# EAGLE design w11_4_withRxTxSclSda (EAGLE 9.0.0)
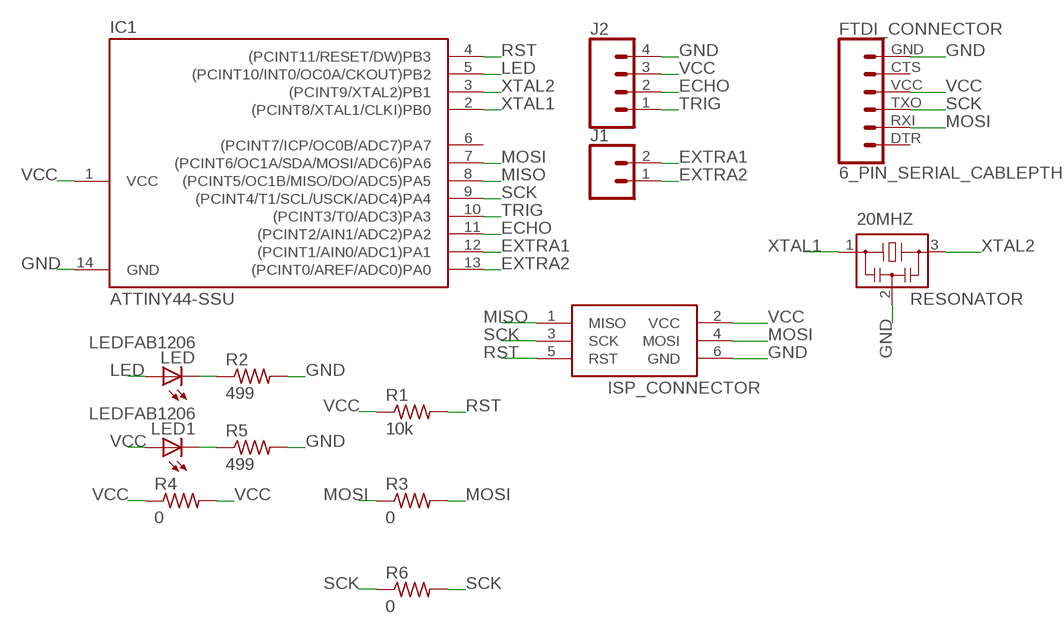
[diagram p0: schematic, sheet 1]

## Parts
20MHZ  RESONATOR  [EFOBM]
FTDI_CONNECTOR  6_PIN_SERIAL_CABLEPTH  [FTDI_BASIC]
IC1  ATTINY44-SSU  [SOIC14]
ISP_CONNECTOR  AVRISP-6  [AVRISP]
J1  CONN_02  [1X02]
J2  CONN_04  [1X04]
LED  LEDFAB1206  [LED1206FAB]
LED1  LEDFAB1206  [LED1206FAB]
R1  10k  RES-US1206FAB  [R1206FAB]
R2  499  RES-US1206FAB  [R1206FAB]
R3  0  RES-US1206FAB  [R1206FAB]
R4  0  RES-US1206FAB  [R1206FAB]
R5  499  RES-US1206FAB  [R1206FAB]
R6  0  RES-US1206FAB  [R1206FAB]

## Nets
ECHO: IC1.11((PCINT2/AIN1/ADC2)PA2) J2.2
EXTRA1: IC1.12((PCINT1/AIN0/ADC1)PA1) J1.2
EXTRA2: IC1.13((PCINT0/AREF/ADC0)PA0) J1.1
GND: 20MHZ.2 FTDI_CONNECTOR.GND IC1.14(GND) ISP_CONNECTOR.6(GND) J2.4 R2.2 R5.2
LED: IC1.5((PCINT10/INT0/OC0A/CKOUT)PB2) LED.1(A)
MISO: IC1.8((PCINT5/OC1B/MISO/DO/ADC5)PA5) ISP_CONNECTOR.1(MISO)
MOSI: FTDI_CONNECTOR.RXI IC1.7((PCINT6/OC1A/SDA/MOSI/ADC6)PA6) ISP_CONNECTOR.4(MOSI) R3.1 R3.2
N$1: LED1.2(C) R5.1
N$5: LED.2(C) R2.1
RST: IC1.4((PCINT11/RESET/DW)PB3) ISP_CONNECTOR.5(RST) R1.2
SCK: FTDI_CONNECTOR.TXO IC1.9((PCINT4/T1/SCL/USCK/ADC4)PA4) ISP_CONNECTOR.3(SCK) R6.1 R6.2
TRIG: IC1.10((PCINT3/T0/ADC3)PA3) J2.1
VCC: FTDI_CONNECTOR.VCC IC1.1(VCC) ISP_CONNECTOR.2(VCC) J2.3 LED1.1(A) R1.1 R4.1 R4.2
XTAL1: 20MHZ.1 IC1.2((PCINT8/XTAL1/CLKI)PB0)
XTAL2: 20MHZ.3 IC1.3((PCINT9/XTAL2)PB1)
Unconnected: FTDI_CONNECTOR.CTS FTDI_CONNECTOR.DTR IC1.6((PCINT7/ICP/OC0B/ADC7)PA7)

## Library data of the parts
20MHZ = fab:RESONATOR
FTDI_CONNECTOR = SparkFun-Connectors:6_PIN_SERIAL_CABLE: 6-pin header connection for use with the "FTDI BASIC" pinout - CABLE SIDE. Also known as "Arduino Serial Program Header". This is used on a design to provide a 6-pin connection point for serial communication usually from a USB cable (D+/D-) to these headers (RX/TX). It also has the remaining pins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
IC1 = fab:ATTINY44
ISP_CONNECTOR = adafruit:AVRISP: AVR ISP HEADER Standard 6 pin header for AVR programming
J1 = SparkFun-Connectors:CONN_02: Multi connection point. Often used as Generic Header-pin footprint for 0.1 inch spaced/style header connections
J2 = SparkFun-Connectors:CONN_04: Multi connection point. Often used as Generic Header-pin footprint for 0.1 inch spaced/style header connections On any of the 0.1 inch spaced packages, you can populate with these: Break Away Headers - Straight (PRT-00116) Break Away Male Headers - Right Angle (PRT-00553) Female Headers (PRT-00115)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; PROD_ID: CONN-09696
LED LED1 = fab:LED: LED
R1-R6 = fab:RES-US: Resistor (US Symbol)

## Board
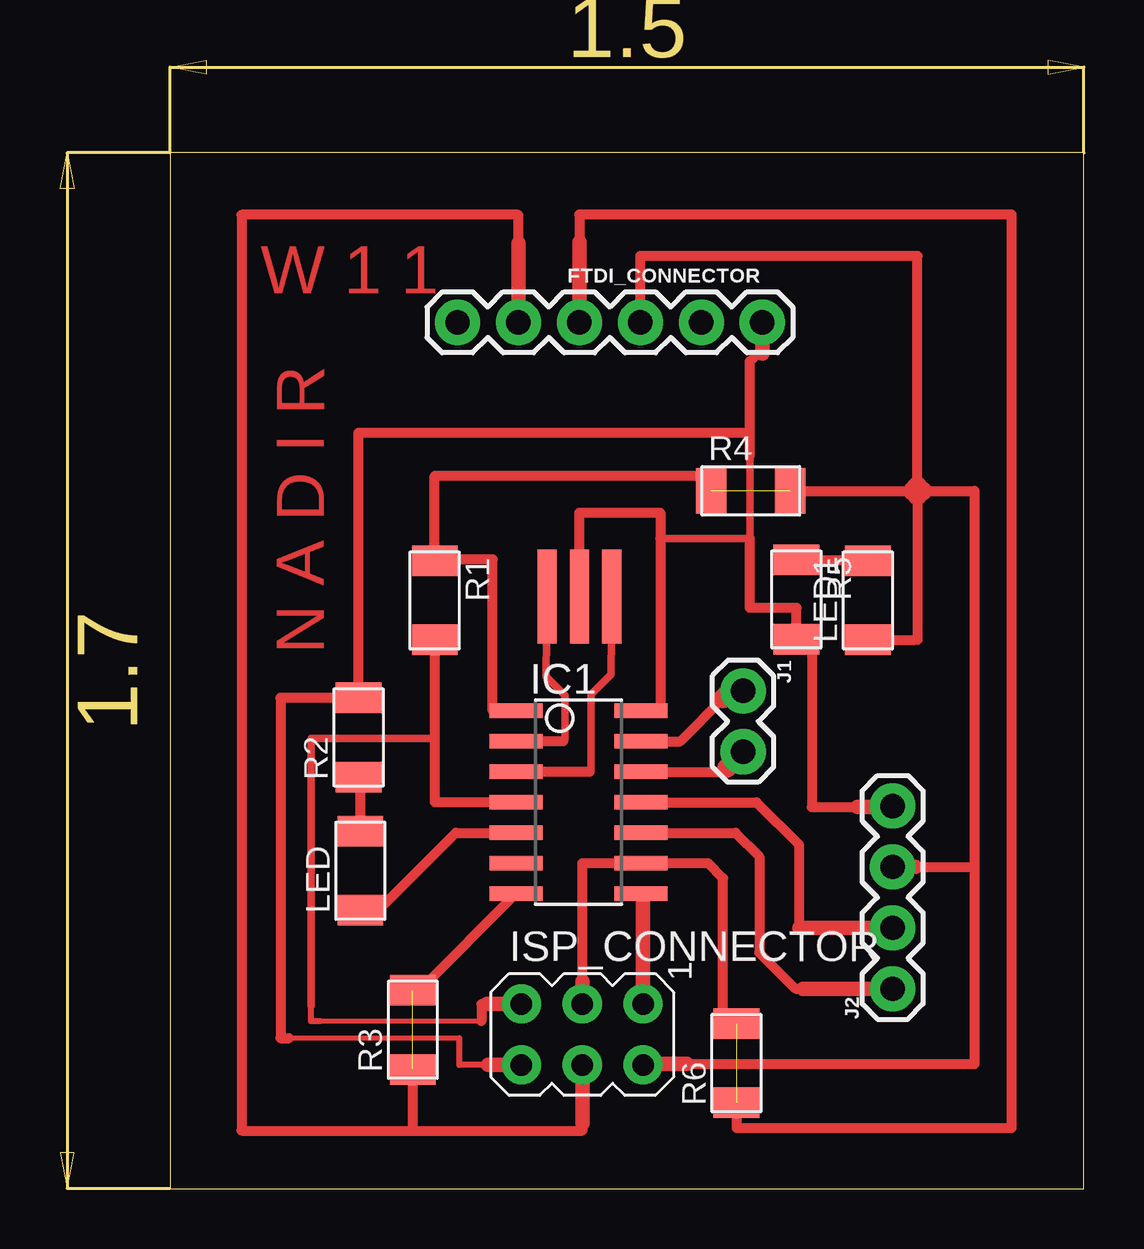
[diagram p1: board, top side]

Size 42.69 x 47.05 mm. Coordinates in mm from the lower left corner, seen from the top.
Outline: 4.59,0 42.69,0 42.69,43.18 4.59,43.18 4.59,0
Copper layers (1*16): Top 0.035mm / dielectric 1.5mm / Bottom 0.035mm
Design rules "default": minimum track width 6mil, minimum drill 0.35mm, track to track 6mil, track to pad 6mil, pad to pad 6mil, via to via 6mil, smd to smd 6mil, copper to edge 40mil, drill to drill 6mil, minimum pad ring 10mil, minimum via ring 8mil, stop-mask expansion 4mil, vias tented up to drill 0mil, thermal gap 10mil

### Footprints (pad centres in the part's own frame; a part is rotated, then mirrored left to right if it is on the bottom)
EFOBM = smd 0.8 x 3.9: 1 -1.35,0; 2 0,0; 3 1.35,0
FTDI_BASIC = drill 1.016 pad 1.88: CTS 10.16,0; DTR 0,0; GND 12.7,0; RXI 2.54,0; TXO 5.08,0; VCC 7.62,0
SOIC14 = smd 0.61 x 2.21: 1 -3.81,-2.603; 2 -2.54,-2.603; 3 -1.27,-2.603; 4 0,-2.603; 5 1.27,-2.603; 6 2.54,-2.603; 7 3.81,-2.603; 8 3.81,2.603; 9 2.54,2.603; 10 1.27,2.603; 11 0,2.603; 12 -1.27,2.603; 13 -2.54,2.603; 14 -3.81,2.603
AVRISP = drill 0.9 pad 1.626: 1 -1.27,2.54; 2 1.27,2.54; 3 -1.27,0; 4 1.27,0; 5 -1.27,-2.54; 6 1.27,-2.54
1X02 = drill 1.016 pad 1.88: 1 0,0; 2 2.54,0
1X04 = drill 1.016 pad 1.88: 1 0,0; 2 2.54,0; 3 5.08,0; 4 7.62,0
LED1206FAB = smd 1.27 x 1.905: 1 -1.651,0; 2 1.651,0
R1206FAB = smd 1.27 x 1.905: 1 -1.651,0; 2 1.651,0

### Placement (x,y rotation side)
20MHZ  21.65,24.69 0 top
FTDI_CONNECTOR  16.57,36.12 0 top
IC1  21.61,16.11 270 top
ISP_CONNECTOR  21.77,6.43 270 top
J1  28.48,20.76 270 top
J2  34.71,8.33 90 top
LED  12.52,13.26 90 top
LED1  33.68,24.53 90 top
R1  15.62,24.53 270 top
R2  12.44,18.81 90 top
R3  14.71,6.63 90 top
R4  28.8,29.09 0 top
R5  30.7,24.57 270 top
R6  28.2,5.24 90 top

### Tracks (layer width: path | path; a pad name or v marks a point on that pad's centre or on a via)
ECHO
  Top 0.406: IC1.11 29.03,16.11 30.82,14.33 30.82,10.87
  Top 0.61: J2.2 30.82,10.87
EXTRA1
  Top 0.406: IC1.12 27.64,17.38 27.8,17.54
  Top 0.813: J1.2 27.8,17.54
EXTRA2
  Top 0.406: IC1.13 25.86,18.65 27.64,20.44
  Top 0.813: J1.1 27.96,20.76 27.64,20.44
GND
  Top 0.203: 16.65,6.27 9.55,6.27 9.43,6.27
  Top 0.254: 17.84,5.16 16.65,5.16 16.65,6.27
  Top 0.305: 25.03,27.11 28.76,27.11 28.76,30.56 28.76,30.92
  Top 0.406: IC1.14 25.03,19.92 25.03,27.11 25.03,28.18 21.65,28.18 20MHZ.2 | 9.55,6.27 9.19,6.27 9.19,20.46 R2.2 12.44,31.51 28.68,31.51 28.76,31.43 | 29.27,35.93 29.27,35 28.76,34.49 28.76,31.43 | 28.76,27.11 28.76,24.21 30.7,24.21 R5.2 31.34,22.92 31.34,15.91 33.24,15.91 | 28.76,30.56 28.76,31.43
  Top 0.61: ISP_CONNECTOR.6 17.84,5.16 | 29.27,34.81 29.27,35 FTDI_CONNECTOR.GND | 33.24,15.91 34.71,15.91 J2.4
LED
  Top 0.406: LED.1 13.25,11.61 16.49,14.84 IC1.5
MISO
  Top 0.61: IC1.8 24.31,12.3 ISP_CONNECTOR.1
MOSI  (1 unrouted)
  Top 0.406: IC1.7 14.98,8.28 R3.2 | R3.1 14.71,2.42 | 21.77,2.74 21.77,2.42 14.71,2.42 | 14.71,2.42 7.56,2.42 7.56,40.6 19.11,40.6 19.11,39.41
  Top 0.61: ISP_CONNECTOR.4 21.77,2.74 | FTDI_CONNECTOR.RXI 19.11,39.41
N$1
  Top 0.406: R5.1 33.64,26.22 LED1.2
N$5
  Top 0.406: LED.2 12.52,17.08 R2.1
RST
  Top 0.203: 17.56,6.99 10.86,6.99
  Top 0.254: 10.86,6.99 10.46,6.99 10.46,7.62
  Top 0.305: 15.62,19.17 15.62,18.81 | 15.62,18.65 15.62,18.77 10.46,18.77 10.46,7.62
  Top 0.406: IC1.4 15.62,16.11 15.62,18.65 15.62,19.17 R1.2 | 17.56,6.99 17.56,7.7 18.36,7.7
  Top 0.61: ISP_CONNECTOR.5 18.36,7.7 17.8,7.7
SCK  (1 unrouted)
  Top 0.406: 21.77,8.65 21.77,13.57 IC1.9 27.01,13.57 27.64,12.94 27.64,6.89 R6.2 | 21.65,39.45 21.65,40.61 39.67,40.61 39.67,2.54 28.2,2.54 R6.1
  Top 0.61: ISP_CONNECTOR.3 21.77,8.65 | 21.65,39.45 FTDI_CONNECTOR.TXO
TRIG
  Top 0.406: IC1.10 28.16,14.84 29.15,13.85 29.15,9.84 30.66,8.33 30.98,8.33
  Top 0.61: 30.98,8.33 J2.1
VCC  (1 unrouted)
  Top 0.406: R4.1 27.14,29.73 15.62,29.73 R1.1 15.62,26.23 18.04,26.23 18.04,19.92 IC1.1 | R4.2 35.54,29.09 35.74,29.09 | LED1.1 35.64,22.88 | 35.64,22.88 35.66,22.9 | 35.94,29.09 38.12,29.09 38.12,13.41 | 26.14,5.2 38.12,5.2 38.12,13.41 | 35.66,13.41 38.12,13.41 | FTDI_CONNECTOR.VCC 24.19,38.89 35.74,38.89 35.74,29.29 | 35.74,28.89 35.74,22.88 35.64,22.88
  Top 0.61: J2.3 35.66,13.41 | 26.14,5.2 24.31,5.2 ISP_CONNECTOR.2
  Top 0.813: 35.74,29.09 35.74,29.29 35.54,29.09 | 35.74,29.09 35.74,28.89 | 35.74,29.09 35.94,29.09
XTAL1
  Top 0.305: 20MHZ.1 20.26,21.35 21.06,20.56 21.06,18.73 20.98,18.65
  Top 0.406: 20.98,18.65 IC1.2 | 20.18,23.5 20MHZ.1
XTAL2
  Top 0.305: 20MHZ.3 22.96,21.43 22.13,20.6 22.13,17.42 22.09,17.38
  Top 0.406: 22.09,17.38 IC1.3

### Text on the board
Top: W 1 1 | N A D I R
